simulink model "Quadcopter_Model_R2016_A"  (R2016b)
settings: Solver=VariableStepAuto  StartTime=0.0  StopTime=10.0  RelTol=1e-3
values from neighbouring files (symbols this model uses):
  g = 9.81    [modelParameters.m]    (also in getMomentOfInertia.m = 9.80665)
  If = 0.511    [modelParameters.m]    (also in thrustDragConstantCalculations.m = [If0; If1; If2; If3]; Kd_error.m = I_0 * sign(rotor_speed_0) + I_1 * rotor_speed_0 + I_2 * roto)
  Jreq = 4.2012e-05    [modelParameters.m]
  Jxx = 0.0218    [modelParameters.m]
  Jyy = 0.0277    [modelParameters.m]
  Jzz = 0.0332    [modelParameters.m]
  Kd = 1.8087e-07    [modelParameters.m]    (also in calcDragConstant.m = ((A'*A)^-1)*A'*b; thrustDragConstantCalculations.m = calcDragConstant(data, Pmin, Pmax, Rm, Kv, Kq, If ))
  Kq = 96.3422    [modelParameters.m]    (also in thrustDragConstantCalculations.m; Kd_error.m)
  Kt = 8.1558*10^-6    (= 8.1558e-06)    [modelParameters.m]    (also in calcThrustConstant.m = ((A'*A)^(-1))*(A'*T); thrustDragConstantCalculations.m = calcThrustConstant(data))
  Kv = 96.3422    [modelParameters.m]    (also in thrustDragConstantCalculations.m; Kd_error.m)
  m = 1.19    [modelParameters.m]
  Pmax = 0.80    (= 0.8)    [modelParameters.m]    (also in thrustDragConstantCalculations.m; Kd_error.m)
  Pmin = 0.40    (= 0.4)    [modelParameters.m]    (also in thrustDragConstantCalculations.m; Kd_error.m)
  rhx = 0.016    [modelParameters.m]
  rhy = 0.016    [modelParameters.m]
  rhz = 0.003    [modelParameters.m]
  Rm = 0.2308    [modelParameters.m]    (also in thrustDragConstantCalculations.m; Kd_error.m)
  Vb = 11.1    [modelParameters.m]    (also in calcDragConstant.m = [data.(6); data.(6); data.(6); data.(6)]; Kd_error.m = data.(6))

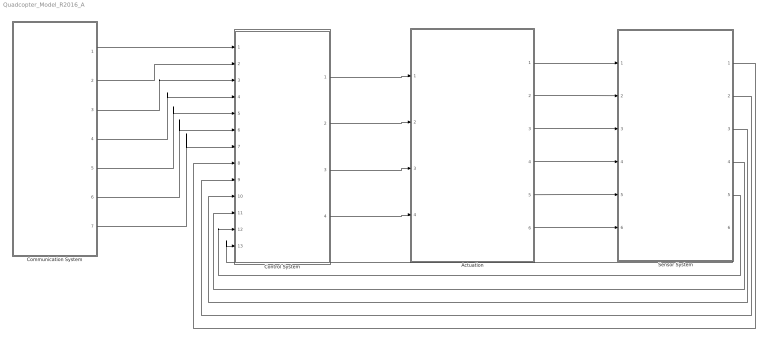
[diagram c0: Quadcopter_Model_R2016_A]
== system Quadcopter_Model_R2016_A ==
  Actuation : Subsystem
  Communication System : Subsystem
  Control System : Subsystem
  Sensor System : Subsystem
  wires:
  Control System/1(Rotor 0 Duty Cycle) -> Actuation/1(Rotor 0 Duty Cycle)
  Sensor System/6(Yaw rate (psi dot)) -> Control System/13(Yaw rate (psi dot))
  Sensor System/5(Roll rate (theta dot)) -> Control System/12(Roll rate (theta dot))
  Sensor System/4(Pitch rate (phi dot)) -> Control System/11(Pitch rate (phi dot))
  Sensor System/3(Yaw (psi)) -> Control System/10(Yaw (psi))
  Sensor System/2(Roll (theta)) -> Control System/9(Roll (theta))
  Sensor System/1(Pitch (phi)) -> Control System/8(Pitch (phi))
  Communication System/1(x_position) -> Control System/1(x position)
  Communication System/2(y_position) -> Control System/2(y position)
  Communication System/3(z_position) -> Control System/3(z position)
  Communication System/4(x_setpoint) -> Control System/4(x setpoint)
  Communication System/5(y_setpoint) -> Control System/5(y setpoint)
  Communication System/6(z_setpoint) -> Control System/6(z setpoint)
  Communication System/7(yaw_setpoint) -> Control System/7("Yaw setpoint ")
  Control System/2(Rotor 1 Duty Cycle) -> Actuation/2(Rotor 1 Duty Cycle)
  Control System/3(Rotor 2 Duty Cycle) -> Actuation/3(Rotor 2 Duty Cycle)
  Control System/4(Rotor 3 Duty Cycle) -> Actuation/4(Rotor 3 Duty Cycle)
  Actuation/1(B_omega) -> Sensor System/1(B_Omega)
  Actuation/2(euler_angles) -> Sensor System/2(euler_angles)
  Actuation/3(B_vo) -> Sensor System/3(B_vo)
  Actuation/4(E_ro) -> Sensor System/4(E_ro)
  Actuation/5(B_vo_dot) -> Sensor System/5(B_vo_dot)
  Actuation/6(B_Fg) -> Sensor System/6(B_Fg)

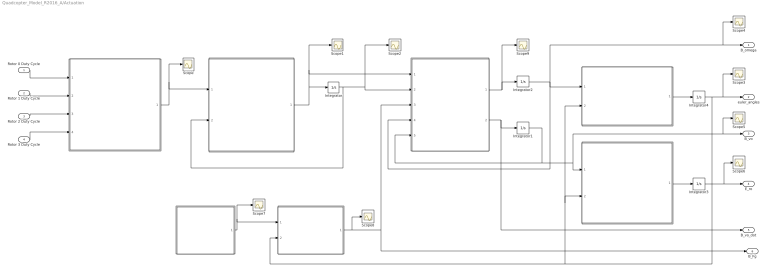
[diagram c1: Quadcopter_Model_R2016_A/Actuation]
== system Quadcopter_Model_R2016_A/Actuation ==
  Rotor 0 Duty Cycle : Inport
  Rotor 1 Duty Cycle : Inport  Port=2
  Rotor 2 Duty Cycle : Inport  Port=3
  Rotor 3 Duty Cycle : Inport  Port=4
  " " : MATLAB Function  TreatAsAtomicUnit=on
  " " : MATLAB Function  TreatAsAtomicUnit=on
  " " : MATLAB Function  TreatAsAtomicUnit=on
  " " : MATLAB Function  TreatAsAtomicUnit=on
  " " : MATLAB Function  TreatAsAtomicUnit=on
  " " : MATLAB Function  TreatAsAtomicUnit=on
  " " : MATLAB Function  TreatAsAtomicUnit=on
  Integrator{,1..3} (4 alike) : Integrator
  Integrator4 : Integrator  ContinuousStateAttributes=['phi' 'theta' 'psi']
  Scope{,1..9} (10 alike) : Scope
  B_omega : Outport
  euler_angles : Outport  Port=2
  B_vo : Outport  Port=3
  E_ro : Outport  Port=4
  B_vo_dot : Outport  Port=5
  B_Fg : Outport  Port=6
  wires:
  Rotor 3 Duty Cycle/1 -> " "/4(rotor_3_duty_cycle)
  Rotor 2 Duty Cycle/1 -> " "/3(rotor_2_duty_cycle)
  Rotor 1 Duty Cycle/1 -> " "/2(rotor_1_duty_cycle)
  Rotor 0 Duty Cycle/1 -> " "/1(rotor_0_duty_cycle)
  " "/1(Vb_eff) -> Scope/1, " "/1(Vb_eff)
  " "/1(angular_acceleration) -> Integrator/1, Scope1/1, " "/1(angular_acceleration)
  Integrator/1 -> Scope2/1, " "/2(angular_velocity), " "/2(angular_velocity)
  " "/1(B_omega_dot) -> Scope9/1, Integrator2/1
  " "/2(B_vo_dot) -> B_vo_dot/1, Integrator1/1
  Integrator2/1 -> Scope4/1, B_omega/1, " "/4(B_omega), " "/1(B_omega)
  Integrator1/1 -> " "/5(B_vo), " "/1(B_vo), B_vo/1, Scope5/1
  " "/1(euler_rates) -> Integrator4/1
  Integrator4/1 -> Scope3/1, euler_angles/1, " "/2(euler_angles), " "/2(euler_angles), " "/2(euler_angles)
  " "/1(E_Fg) -> Scope7/1, " "/1(E_Fg)
  " "/1(E_ro) -> Integrator3/1
  Integrator3/1 -> Scope6/1, E_ro/1
  " "/1(B_Fg) -> Scope8/1, B_Fg/1, " "/3(B_Fg)

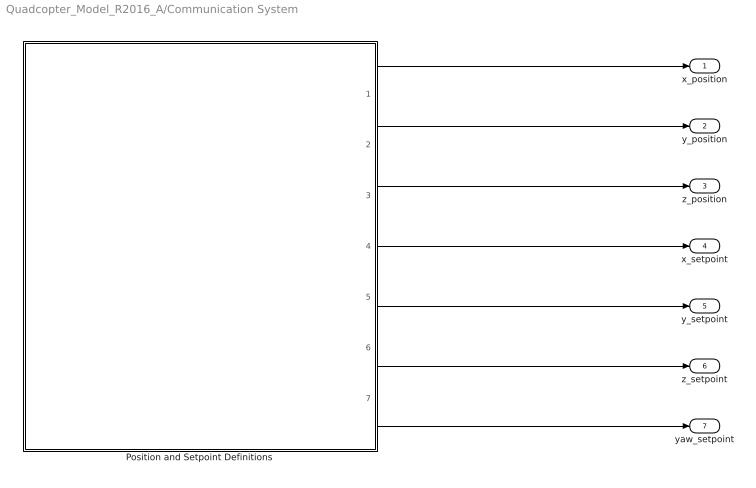
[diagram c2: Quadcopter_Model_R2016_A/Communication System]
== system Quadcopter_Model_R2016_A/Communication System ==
  Position and Setpoint Definitions : MATLAB Function  TreatAsAtomicUnit=on
  x_position : Outport
  y_position : Outport  Port=2
  z_position : Outport  Port=3
  x_setpoint : Outport  Port=4
  y_setpoint : Outport  Port=5
  z_setpoint : Outport  Port=6
  yaw_setpoint : Outport  Port=7
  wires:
  Position and Setpoint Definitions/7(yaw_setpoint) -> yaw_setpoint/1
  Position and Setpoint Definitions/6(z_setpoint) -> z_setpoint/1
  Position and Setpoint Definitions/5(y_setpoint) -> y_setpoint/1
  Position and Setpoint Definitions/4(x_setpoint) -> x_setpoint/1
  Position and Setpoint Definitions/3(z_position) -> z_position/1
  Position and Setpoint Definitions/2(y_position) -> y_position/1
  Position and Setpoint Definitions/1(x_position) -> x_position/1

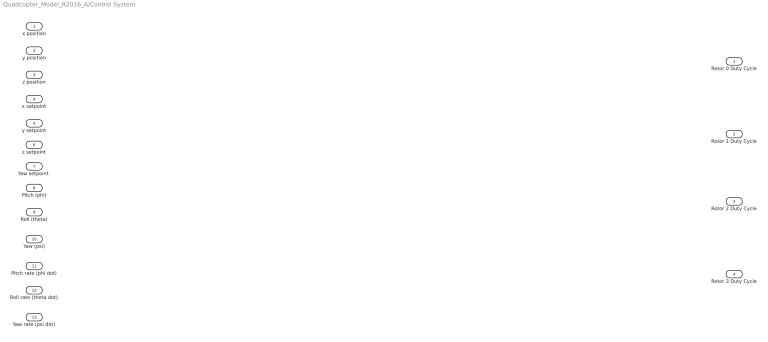
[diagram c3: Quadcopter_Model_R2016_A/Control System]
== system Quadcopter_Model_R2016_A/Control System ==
  x position : Inport
  y position : Inport  Port=2
  z position : Inport  Port=3
  x setpoint : Inport  Port=4
  y setpoint : Inport  Port=5
  z setpoint : Inport  Port=6
  "Yaw setpoint " : Inport  Port=7
  Pitch (phi) : Inport  Port=8
  Roll (theta) : Inport  Port=9
  Yaw (psi) : Inport  Port=10
  Pitch rate (phi dot) : Inport  Port=11
  Roll rate (theta dot) : Inport  Port=12
  Yaw rate (psi dot) : Inport  Port=13
  Rotor 0 Duty Cycle : Outport
  Rotor 1 Duty Cycle : Outport  Port=2
  Rotor 2 Duty Cycle : Outport  Port=3
  Rotor 3 Duty Cycle : Outport  Port=4

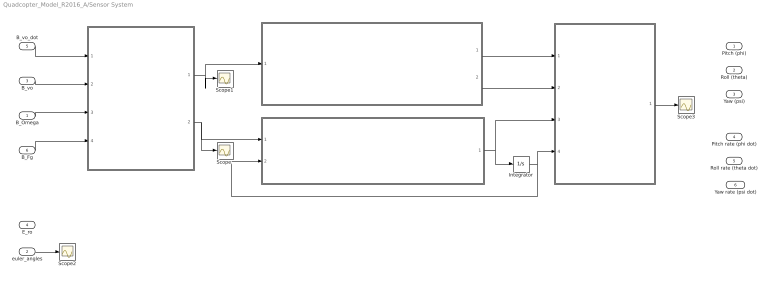
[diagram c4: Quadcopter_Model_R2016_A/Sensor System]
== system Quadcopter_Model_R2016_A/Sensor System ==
  B_Omega : Inport
  euler_angles : Inport  Port=2
  B_vo : Inport  Port=3
  E_ro : Inport  Port=4
  B_vo_dot : Inport  Port=5
  B_Fg : Inport  Port=6
  " " : MATLAB Function  TreatAsAtomicUnit=on
  " " : Subsystem
  " " : MATLAB Function  TreatAsAtomicUnit=on
  " " : MATLAB Function  TreatAsAtomicUnit=on
  Integrator : Integrator
  Scope{,1..3} (4 alike) : Scope
  Pitch (phi) : Outport
  Roll (theta) : Outport  Port=2
  Yaw (psi) : Outport  Port=3
  Pitch rate (phi dot) : Outport  Port=4
  Roll rate (theta dot) : Outport  Port=5
  Yaw rate (psi dot) : Outport  Port=6
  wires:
  " "/1(accelerometer) -> " "/1(accel_reading), Scope1/1
  " "/2(gyroscope) -> Scope/1, " "/1(gyro_reading)
  B_vo_dot/1 -> " "/1(B_vo_dot)
  B_vo/1 -> " "/2(B_vo)
  B_Omega/1 -> " "/3(B_Omega)
  B_Fg/1 -> " "/4(B_Fg)
  " "/1(euler_rates_IMU) -> Integrator/1, " "/3(euler_rates_IMU)
  " "/2(accel_roll) -> " "/2(accel_roll)
  " "/1(accel_pitch) -> " "/1(accel_pitch)
  euler_angles/1 -> Scope2/1
  " "/1(euler_angles_IMU) -> Scope3/1
  Integrator/1 -> " "/2(euler_angles_IMU), " "/4(prev_euler_angles_IMU)

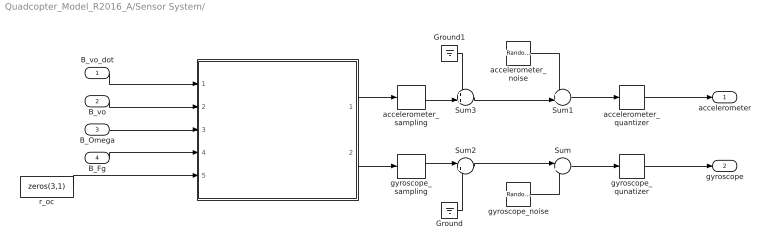
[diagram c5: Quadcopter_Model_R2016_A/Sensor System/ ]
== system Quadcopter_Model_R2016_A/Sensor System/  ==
  B_vo_dot : Inport
  B_vo : Inport  Port=2
  B_Omega : Inport  Port=3
  B_Fg : Inport  Port=4
  " " : MATLAB Function  TreatAsAtomicUnit=on
  Ground : Ground
  Ground1 : Ground
  Sum : Sum  Inputs=|++
  Sum1 : Sum  Inputs=++|
  Sum2 : Sum  Inputs=|++
  Sum3 : Sum  Inputs=++|
  accelerometer_noise : RandomNumber  Mean=zeros(3,1)  Variance=[ 3e-7 ; 3.3e-7 ; 7.2e-7 ]  Seed=[0,1,2]  SampleTime=6.1e-3
  accelerometer_quantizer : Quantizer  QuantizationInterval=2.4400e-04
  accelerometer_sampling : ZeroOrderHold  SampleTime=6.1e-3
  gyroscope_noise : RandomNumber  Mean=zeros(3,1)  Variance=[ 2.2e-8 ; 1.1e-7 ; 2.4e-8 ]  Seed=[0,1,2]  SampleTime=6.1e-3
  gyroscope_qunatizer : Quantizer  QuantizationInterval=1.1e-3
  gyroscope_sampling : ZeroOrderHold  SampleTime=6.1e-3
  r_oc : Constant  Value=zeros(3,1)
  accelerometer : Outport
  gyroscope : Outport  Port=2
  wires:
  gyroscope_qunatizer/1 -> gyroscope/1
  accelerometer_quantizer/1 -> accelerometer/1
  accelerometer_noise/1 -> Sum1/1
  Sum/1 -> gyroscope_qunatizer/1
  Sum2/1 -> Sum/1
  Sum3/1 -> Sum1/2
  " "/2(gyroReading) -> gyroscope_sampling/1
  gyroscope_noise/1 -> Sum/2
  " "/1(accelReading) -> accelerometer_sampling/1
  Sum1/1 -> accelerometer_quantizer/1
  gyroscope_sampling/1 -> Sum2/1
  accelerometer_sampling/1 -> Sum3/2
  Ground/1 -> Sum2/2
  Ground1/1 -> Sum3/1
  B_vo_dot/1 -> " "/1(B_vo_dot)
  B_vo/1 -> " "/2(B_vo)
  B_Omega/1 -> " "/3(B_Omega)
  B_Fg/1 -> " "/4(B_Fg)
  r_oc/1 -> " "/5(r_oc)

== matlab function Quadcopter_Model_R2016_A/Actuation/



 ==
function E_Fg = gravity(  m, g)

E_Fg = [0; 0; m*g];

== matlab function Quadcopter_Model_R2016_A/Actuation/






 ==
function E_ro  = linear_body_earth_conversion(B_vo, euler_angles)

euler_rates = zeros(3,1);
E_ro = zeros(3,1);

phi = euler_angles(1);
theta = euler_angles(2);
psi = euler_angles(3);

Leb = [cos(theta)*cos(psi), sin(phi)*sin(theta)*cos(psi)-cos(phi)*sin(psi), cos(phi)*sin(theta)*cos(psi)+sin(phi)*sin(psi); ...
       cos(theta)*sin(psi), sin(phi)*sin(theta)*sin(psi)+cos(phi)*cos(psi), cos(phi)*sin(theta)*sin(psi)-sin(phi)*cos(psi); ...
           -sin(theta)    ,                sin(phi)*cos(theta)            ,                 cos(phi)*cos(theta)           ];

E_ro = Leb * B_vo;

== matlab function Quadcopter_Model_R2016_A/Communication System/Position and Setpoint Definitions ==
function [x_position, y_position, z_position, x_setpoint,...
    y_setpoint, z_setpoint, yaw_setpoint]= positionAndSetpointDefinitions

x_position = 0;
y_position = 0;
z_position = 0;
x_setpoint = 0;
y_setpoint = 0;
z_setpoint = 0;
yaw_setpoint = 0;

end

== matlab function Quadcopter_Model_R2016_A/Actuation/

 ==
function Vb_eff   = ESC(rotor_0_duty_cycle, rotor_1_duty_cycle, rotor_2_duty_cycle, rotor_3_duty_cycle, Pmin, Pmax, Vb)

% Define u_Pi for each of the rotors
u_P0 = (rotor_0_duty_cycle/100 - Pmin) / (Pmax - Pmin);
u_P1 = (rotor_1_duty_cycle/100 - Pmin) / (Pmax - Pmin);
u_P2 = (rotor_2_duty_cycle/100 - Pmin) / (Pmax - Pmin);
u_P3 = (rotor_3_duty_cycle/100 - Pmin) / (Pmax - Pmin);

% Determine the effective battery voltage from each ESC
Vb_eff_0 = u_P0 * Vb;
Vb_eff_1 = u_P1 * Vb;
Vb_eff_2 = u_P2 * Vb;
Vb_eff_3 = u_P3 * Vb;

Vb_eff = [Vb_eff_0, Vb_eff_1, Vb_eff_2, Vb_eff_3];

== matlab function Quadcopter_Model_R2016_A/Actuation/
 ==
function angular_acceleration  = motor(Vb_eff, angular_velocity, Rm, Kv, Kq, Kd, If, Jreq)

angular_acceleration = zeros(1,4);

% Define each motors effective battery voltage
Vb_eff_0 = Vb_eff(1);
Vb_eff_1 = Vb_eff(2);
Vb_eff_2 = Vb_eff(3);
Vb_eff_3 = Vb_eff(4);

% Determine the angular velocity of each rotor from feedback
w_0 = angular_velocity(1);
w_1 = angular_velocity(2);
w_2 = angular_velocity(3);
w_3 = angular_velocity(4);

% Determine angular acceleration of each rotor
w_0_dot = 1/(Jreq*Rm*Kq) * Vb_eff_0 - 1/(Jreq*Rm*Kq*Kv) * w_0 - 1/(Jreq*Kq)*If - (Kd/Jreq) * w_0^2;
w_1_dot = 1/(Jreq*Rm*Kq) * Vb_eff_1 - 1/(Jreq*Rm*Kq*Kv) * w_1 - 1/(Jreq*Kq)*If - (Kd/Jreq) * w_1^2;
w_2_dot = 1/(Jreq*Rm*Kq) * Vb_eff_2 - 1/(Jreq*Rm*Kq*Kv) * w_2 - 1/(Jreq*Kq)*If - (Kd/Jreq) * w_2^2;
w_3_dot = 1/(Jreq*Rm*Kq) * Vb_eff_3 - 1/(Jreq*Rm*Kq*Kv) * w_3 - 1/(Jreq*Kq)*If - (Kd/Jreq) * w_3^2;

angular_acceleration = [w_0_dot, w_1_dot, w_2_dot, w_3_dot];

== matlab function Quadcopter_Model_R2016_A/Actuation/







 ==
function [B_omega_dot, B_vo_dot]= rotor(angular_acceleration, angular_velocity, B_Fg, B_omega, B_vo, m, Kt, Kd, rhx, rhy, rhz, Jreq, Jxx, Jyy, Jzz)

B_vo_dot = zeros(3,1);
B_omega_dot = zeros(3,1);

% Create J vector
J = [Jxx,  0 ,  0 ; ...
      0 , Jyy,  0 ; ...
      0 ,  0 , Jzz;];

% Create r_hi vector
rh_0 = [-rhx; rhy; rhz];
rh_1 = [rhx; rhy; rhz];
rh_2 = [-rhx; -rhy; rhz];
rh_3 = [rhx; -rhy; rhz];

% Define vector from body frame origin to center of mass
br_oc = [0; 0; 0];

% Define 3x3 Identity Matrix
I = eye(3);

% Create gamma vectors
gamma_Ti = [0; 0; -1];
gamma_omega_03 = [0; 0; -1];  %Rotors 0 and 3 use this gamma_omega vector
gamma_omega_12 = [0; 0; 1]; %Rotors 1 and 2 use this gamma_omega vector

% Define angular velocities for each rotor
w_0 = angular_velocity(1);
w_1 = angular_velocity(2);
w_2 = angular_velocity(3);
w_3 = angular_velocity(4);

% Define angular acceleration for each rotor
w_0_dot = angular_acceleration(1);
w_1_dot = angular_acceleration(2);
w_2_dot = angular_acceleration(3);
w_3_dot = angular_acceleration(4);

% Define the rotor force in the z-direction from each rotor
B_Fr_0 = Kt * w_0 * w_0 * gamma_Ti;
B_Fr_1 = Kt * w_1 * w_1 * gamma_Ti;
B_Fr_2 = Kt * w_2 * w_2 * gamma_Ti;
B_Fr_3 = Kt * w_3 * w_3 * gamma_Ti;

% Sum up the rotor forces in the z-direction from each vector to get the
% total body force in the z-direction
B_Fr = B_Fr_0 + B_Fr_1 + B_Fr_2 + B_Fr_3;

% Define the in-plane drag and induced torque produced by each rotor
 B_Q_d0 = -1 * Kd * w_0 * w_0 * gamma_omega_03;
 B_Q_d1 = -1 * Kd * w_1 * w_1 * gamma_omega_12;
 B_Q_d2 = -1 * Kd * w_2 * w_2 * gamma_omega_12;
 B_Q_d3 = -1 * Kd * w_3 * w_3 * gamma_omega_03;

% Sum up the total in-plane drag and induced torque to get the total
% in-plane drag and induced torque on the body
B_Q_d = B_Q_d0 + B_Q_d1 + B_Q_d2 + B_Q_d3;

% Define the force lever arm torque created from the force produced by each
% rotor in the z-direction
B_Q_F0 = cross( rh_0, B_Fr_0 );
B_Q_F1 = cross( rh_1, B_Fr_1 );
B_Q_F2 = cross( rh_2, B_Fr_2 );
B_Q_F3 = cross( rh_3, B_Fr_3 );

B_Q_F = B_Q_F0 + B_Q_F1 + B_Q_F2 + B_Q_F3;

%Define the change in angular momentum torque produced by each rotor 
B_Q_L0 = -1 * Jreq * ( cross(B_omega, w_0 * gamma_omega_03) + w_0_dot * gamma_omega_03 );
B_Q_L1 = -1 * Jreq * ( cross(B_omega, w_1 * gamma_omega_12) + w_1_dot * gamma_omega_12 ); 
B_Q_L2 = -1 * Jreq * ( cross(B_omega, w_2 * gamma_omega_12) + w_2_dot * gamma_omega_12 ); 
B_Q_L3 = -1 * Jreq * ( cross(B_omega, w_3 * gamma_omega_03) + w_3_dot * gamma_omega_03 );

% Sum up the total change in angular momentum torque produced by each rotor
B_Q_L = B_Q_L0 + B_Q_L1 + B_Q_L2 + B_Q_L3;

% Define the total rotor system torque as the sum of the in-plane drag and
% induced torque, force lever arm torque, and change in angular momentum
% torques
B_Q = B_Q_d + B_Q_F + B_Q_L;

% Define the body forces in the z-direction from each vector to get the
% total body force in the z-direction
B_F = B_Fr + B_Fg; 

% Define the body frame linear velocities
B_vo_dot = (m*I)^(-1) * ( B_F - cross( B_omega, m*(B_vo + cross(B_omega, br_oc)) ) );

% Define the body frame angular velocities
B_omega_dot = J ^(-1) * ( B_Q - cross(B_omega, J * B_omega) - cross(br_oc, B_F) );

== matlab function Quadcopter_Model_R2016_A/Actuation/














 ==
function euler_rates = angular_body_earth_conversion(B_omega, euler_angles)

euler_rates = zeros(3,1);

phi = euler_angles(1);
theta = euler_angles(2);

Aeb = [1, sin(phi)*tan(theta), cos(phi)*tan(theta); ...
       0,     cos(phi)       ,        -sin(phi)   ; ...
       0,  sin(phi)/cos(theta), cos(phi)/cos(theta)];

   
euler_rates = Aeb * B_omega;

== matlab function Quadcopter_Model_R2016_A/Actuation/






















 ==
function B_Fg  = linear_earth_body_conversion(E_Fg, euler_angles)

euler_rates = zeros(3,1);
B_Fg = zeros(3,1);

phi = euler_angles(1);
theta = euler_angles(2);
psi = euler_angles(3);

Lbe = [             cos(theta)*cos(psi)              ,          cos(theta)*sin(psi)                  ,     -sin(theta)    ; ...
       sin(phi)*sin(theta)*cos(psi)-cos(phi)*sin(psi), sin(phi)*sin(theta)*sin(psi)+cos(phi)*cos(psi), sin(phi)*cos(theta); ...
       cos(phi)*sin(theta)*cos(psi)+sin(phi)*sin(psi), cos(phi)*sin(theta)*sin(psi)-sin(phi)*cos(psi), cos(phi)*cos(theta)];

B_Fg = Lbe * E_Fg;

== matlab function Quadcopter_Model_R2016_A/Sensor System/







 ==
function euler_angles_IMU  = complimentaryFilter(accel_pitch, accel_roll, euler_rates_IMU, prev_euler_angles_IMU)

LOOP_TIME = 5*10^-3;

phi = prev_euler_angles_IMU(1);
theta = prev_euler_angles_IMU(2);
psi = 0;

phi_dot = euler_rates_IMU(1);
theta_dot = euler_rates_IMU(2);

phi = 0.98 * ( phi + theta_dot * LOOP_TIME ) + 0.02 * accel_pitch;
theta = 0.98 * ( theta + phi_dot * LOOP_TIME ) + 0.02 * accel_roll;

euler_angles_IMU = [phi; theta; psi];

== matlab function Quadcopter_Model_R2016_A/Sensor System/









/






 ==
function [accelReading,gyroReading] = idealIMU(B_vo_dot, B_vo, B_Omega, B_Fg, r_oc, g, m)
%#codegen
B_g = B_Fg/m;

a = B_vo_dot + cross(B_Omega,B_vo) ; % body frame acceleration 

accelReading = (a - B_g)/g ; % accelerometer reading (ideal)

gyroReading = B_Omega ; % gyroscope reading (ideal) 

end

== matlab function Quadcopter_Model_R2016_A/Sensor System/











 ==
function [accel_pitch, accel_roll] = getPitchAndRoll(accel_reading)

x_accel = accel_reading(1);
y_accel = accel_reading(2);
z_accel = accel_reading(3);

accel_pitch = atan( x_accel / sqrt( y_accel^2 + z_accel^2 ) );
accel_roll = (-1) * atan( y_accel / sqrt( x_accel^2 + z_accel^2 ) );

== matlab function Quadcopter_Model_R2016_A/Sensor System/














 ==
function euler_rates_IMU = angular_body_earth_conversion(gyro_reading, euler_angles_IMU)

phi = euler_angles_IMU(1);
theta = euler_angles_IMU(2);

Aeb = [1, sin(phi)*tan(theta), cos(phi)*tan(theta); ...
       0,     cos(phi)       ,        -sin(phi)   ; ...
       0,  sin(phi)/cos(theta), cos(phi)/cos(theta)];

   
euler_rates_IMU = Aeb * gyro_reading;
